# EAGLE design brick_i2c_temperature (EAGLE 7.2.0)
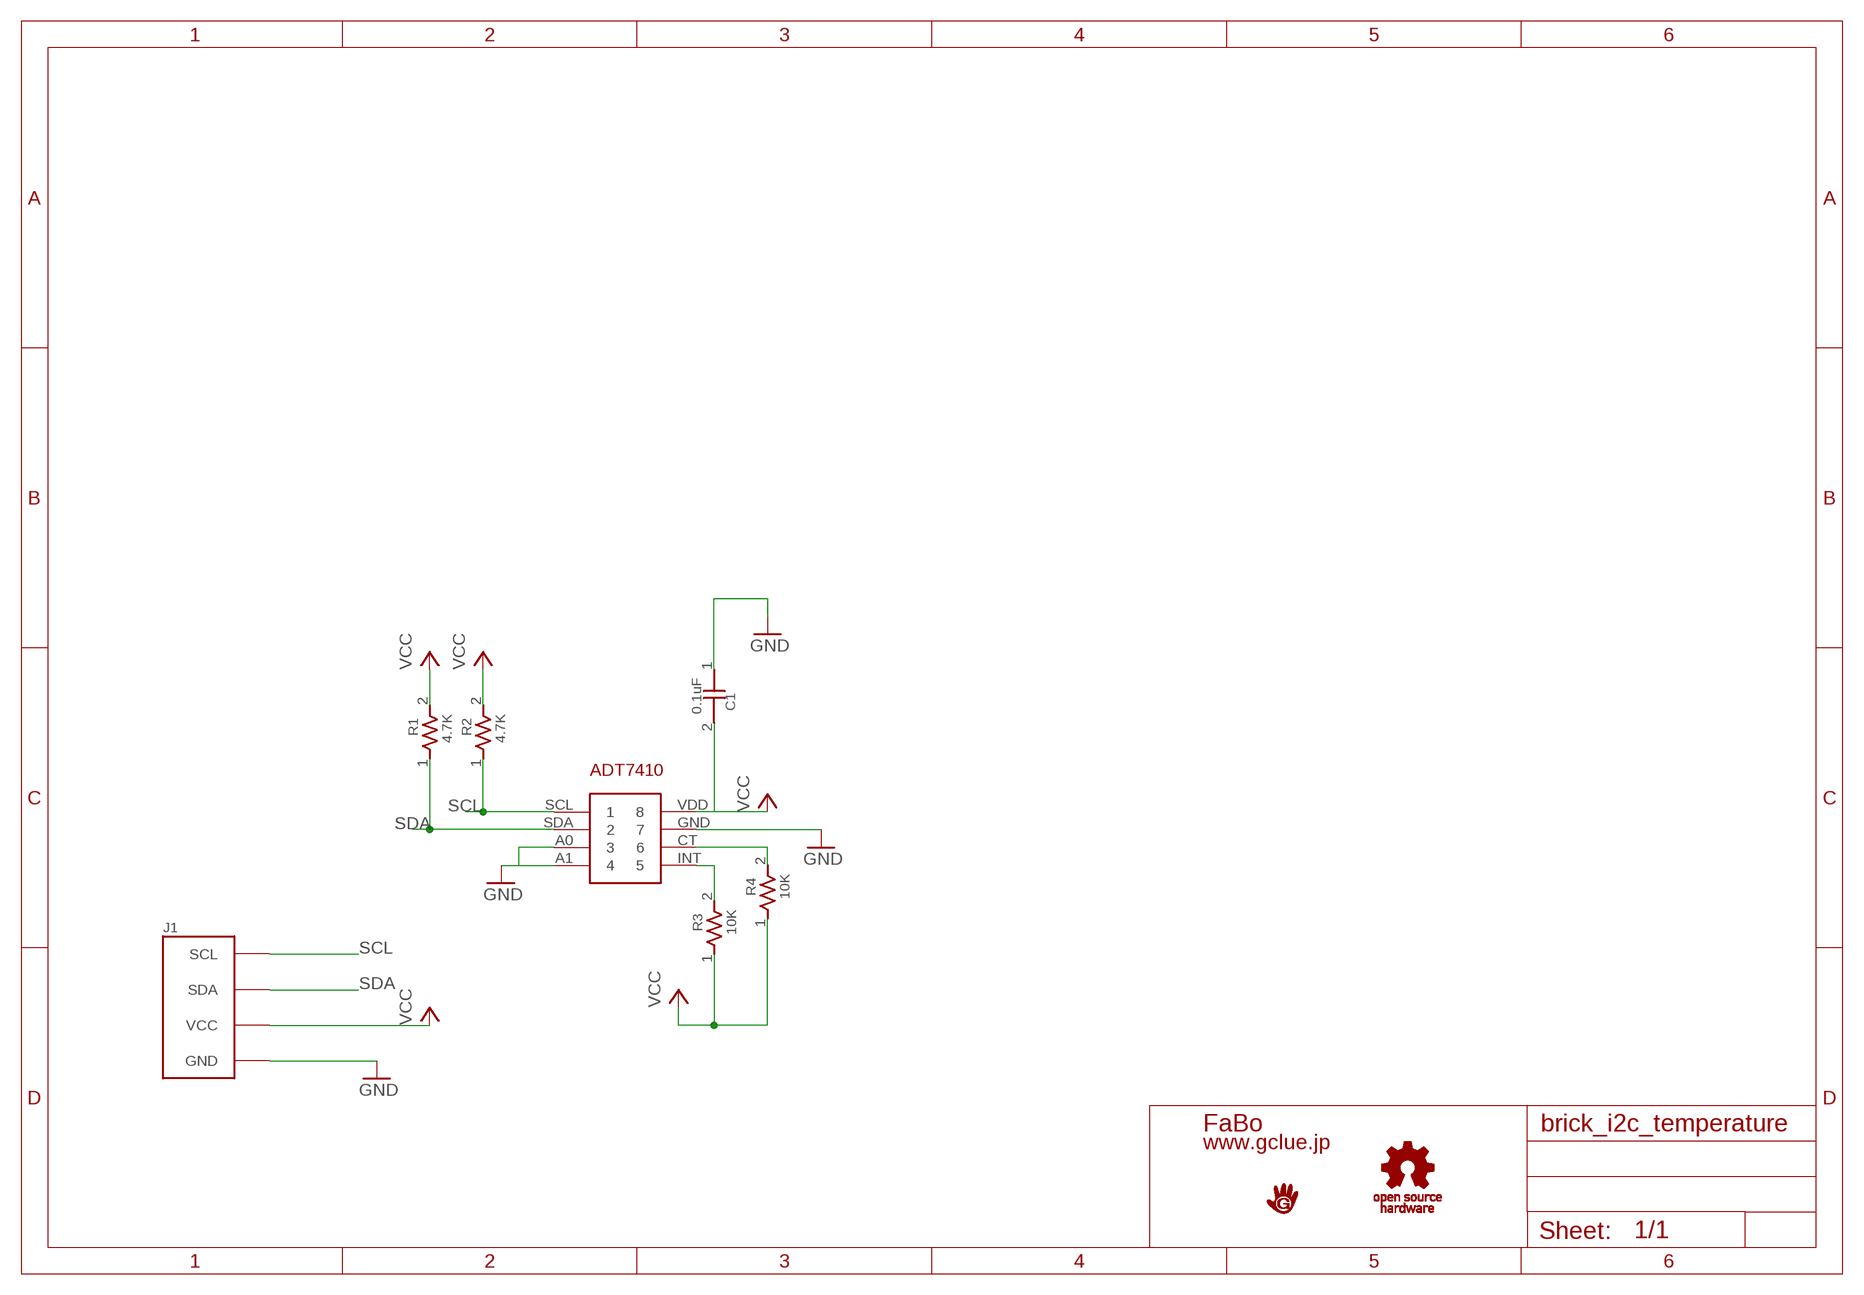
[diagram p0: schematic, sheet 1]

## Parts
C1  0.1uF  CAPACITOR0603  [0603]
J1  BRICK_I2C  [BRICK_I2C]
R1  4.7K  RESISTOR0603  [0603]
R2  4.7K  RESISTOR0603  [0603]
R3  10K  RESISTOR0603  [0603]
R4  10K  RESISTOR0603  [0603]
U$1  I2C-ADT7410  [I2C-ADT7410]
U$3  LOGO_GCLUE-M  [LOGO_GCLUE_M]
U$4  LOGO_OSHW_T-M  [LOGO_OSHW_T_M]

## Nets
GND: C1.1 J1.GND U$1.A0 U$1.A1 U$1.GND
N$2: R3.2 U$1.INT
N$3: R4.2 U$1.CT
SCL: J1.SCL R2.1 U$1.SCL
SDA: J1.SDA R1.1 U$1.SDA
VCC: C1.2 J1.VCC R1.2 R2.2 R3.1 R4.1 U$1.VDD

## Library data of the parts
C1 = GClue-Capacitor:CAPACITOR
J1 = gclue:BRICK_I2C: FaBo Brick 4pin(I2C)
R1-R4 = GClue-Resistors:RESISTOR
U$1 = gclue:I2C-ADT7410
U$3 = gclue:LOGO_GCLUE
U$4 = gclue:LOGO_OSHW_T

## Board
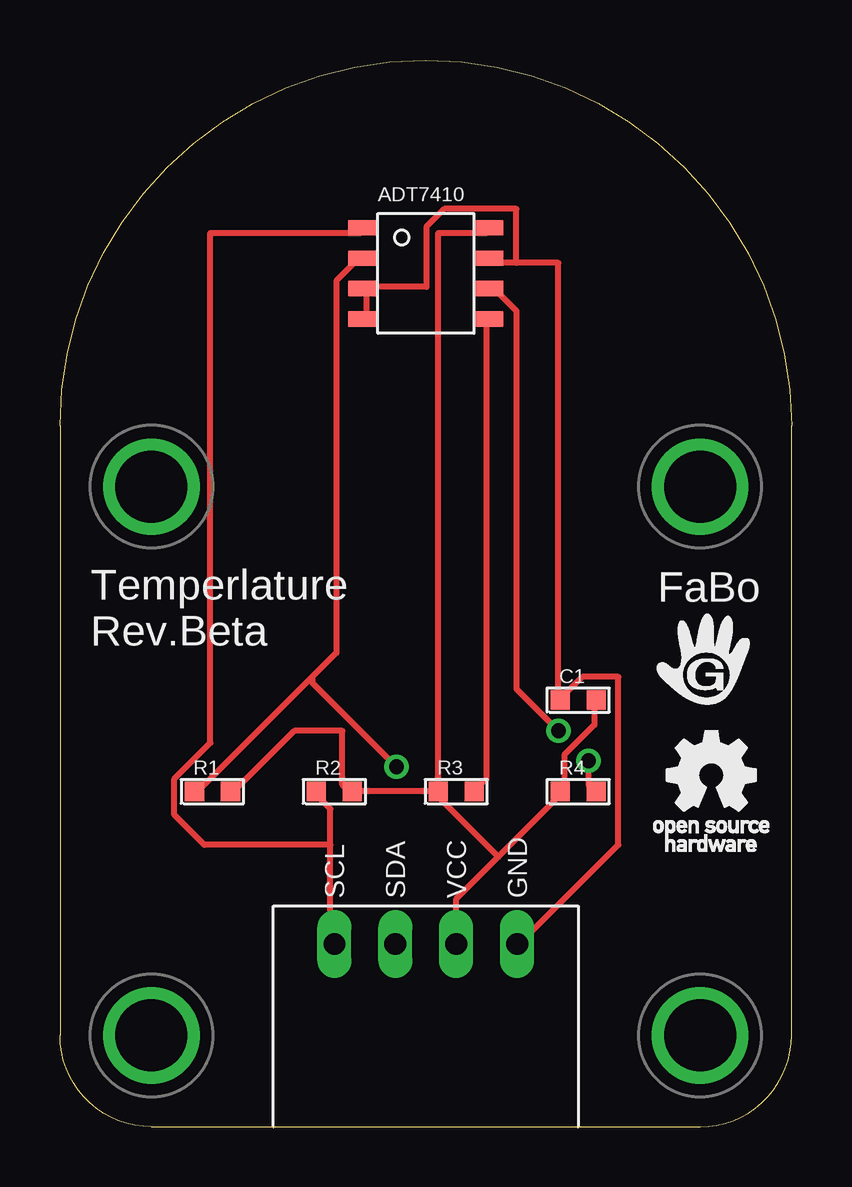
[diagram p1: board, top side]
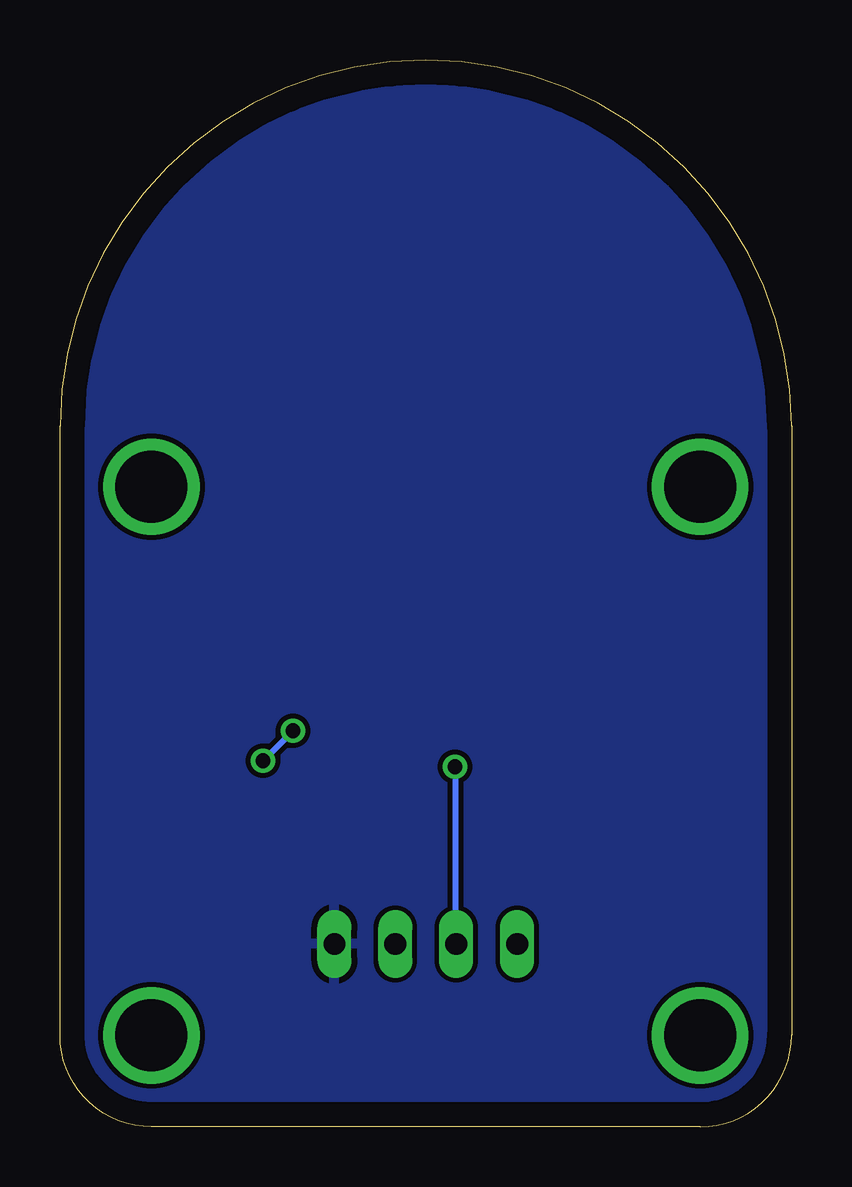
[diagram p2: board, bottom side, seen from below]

Size 30.48 x 44.45 mm. Coordinates in mm from the lower left corner, seen from the top.
Copper layers (1*16): Top 0.035mm / dielectric 1.5mm / Bottom 0.035mm
Design rules "default": minimum track width 10mil, minimum drill 24mil, track to track 8mil, track to pad 8mil, pad to pad 8mil, via to via 8mil, smd to smd 8mil, copper to edge 40mil, drill to drill 8mil, minimum pad ring 10mil, minimum via ring 8mil, stop-mask expansion 4mil, vias tented up to drill 0mil, thermal gap 10mil

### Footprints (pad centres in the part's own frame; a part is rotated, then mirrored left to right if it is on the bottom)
0603 = smd 0.8 x 0.8: 1 -0.75,0; 2 0.75,0
BRICK_I2C = drill 0.9 long: GND 3.81,-11.43; SCL -3.81,-11.43; SDA -1.27,-11.43; VCC 1.27,-11.43 | drill 3 pad 3.81: P$5 -11.43,7.62; P$6 11.43,7.62; P$7 -11.43,-15.24; P$8 11.43,-15.24
I2C-ADT7410 = smd 1.27 x 0.635: A0 -2.6,-0.635; A1 -2.6,-1.905; CT 2.6,-0.635; GND 2.6,0.635; INT 2.6,-1.905; SCL -2.6,1.905; SDA -2.6,0.635; VDD 2.6,1.905

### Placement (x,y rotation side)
C1  21.59,17.78 0 top
J1  15.24,19.05 0 top
R1  6.35,13.97 0 top
R2  11.43,13.97 0 top
R3  16.51,13.97 0 top
R4  21.59,13.97 0 top
U$1  15.24,35.56 0 top
U$3  26.77,19.5 0 top
U$4  27.27,14 0 top

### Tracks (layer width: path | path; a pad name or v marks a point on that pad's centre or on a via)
GND
  Top 0.254: U$1.A1 12.77,33.75 12.77,34.75 U$1.A0 12.77,35 15.27,35 15.27,37.5 16.02,38.25 19.02,38.25 19.02,36 | J1.GND 19.27,7.75 23.27,11.75 23.27,18.75 21.77,18.75 21.02,18 C1.1 20.77,18 20.77,36 19.02,36 | 19.02,36 18.02,36 U$1.GND
  pour Bottom: 0,44.45 30.48,44.45 30.48,0 0,0
N$2
  Top 0.254: R3.2 17.27,14 17.77,14.5 17.77,33.5 U$1.INT
N$3  (via drill 0.61)
  Top 0.254: v22.02,15.25 22.02,14.25 22.27,14 R4.2 | v20.77,16.5 19.02,18.25 19.02,34 18.02,35 U$1.CT
  Bottom 0.254: v20.77,16.5 v22.02,15.25
SCL
  Top 0.254: 11.27,11.75 11.27,7.75 J1.SCL | 11.27,11.75 11.27,13.25 10.77,13.75 R2.1 | 11.27,11.75 6.02,11.75 4.77,13 4.77,14.5 6.27,16 6.27,37.25 12.52,37.25 U$1.SCL
SDA  (via drill 0.61)
  Top 0.254: 10.52,18.75 11.52,19.75 11.52,35.25 12.52,36.25 U$1.SDA | 10.52,18.75 5.77,14 R1.1 | v14.02,15 10.52,18.5 10.52,18.75
  Bottom 0.254: v14.02,15 14.02,7.75 J1.SDA
VCC
  Top 0.254: C1.2 22.27,17.75 22.27,16.75 21.02,15.5 21.02,14 R4.1 20.77,13.75 18.27,11.25 | 18.27,11.25 16.52,9.5 16.52,7.75 J1.VCC | R1.2 7.27,14 9.77,16.5 11.77,16.5 11.77,14.25 12.02,14 R2.2 12.27,14 15.52,14 R3.1 | U$1.VDD 17.77,37.25 15.77,37.25 15.77,14 R3.1 | 18.27,11.25 15.77,13.75 R3.1

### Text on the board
tPlace: FaBo | Temperlature / Rev.Beta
